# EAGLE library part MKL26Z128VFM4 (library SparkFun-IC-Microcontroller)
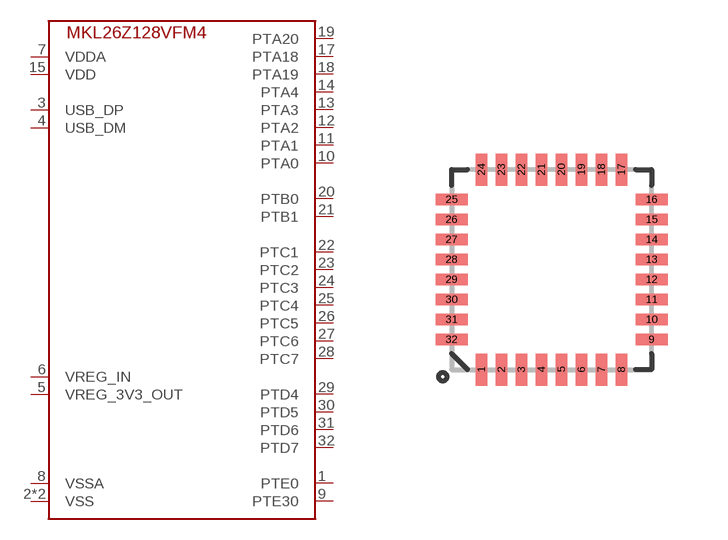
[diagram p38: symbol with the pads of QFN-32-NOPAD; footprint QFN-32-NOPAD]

Designator prefix -

## MKL26Z128VFM4 (PROD_ID: IC-15168)  [QFN-32-NOPAD]
1  PTE0
2  VSS
3  USB_DP
4  USB_DM
5  VREG_3V3_OUT
6  VREG_IN
7  VDDA
8  VSSA
9  PTE30
10  PTA0
11  PTA1
12  PTA2
13  PTA3
14  PTA4
15  VDD
16  VSS
17  PTA18
18  PTA19
19  PTA20
20  PTB0
21  PTB1
22  PTC1
23  PTC2
24  PTC3
25  PTC4
26  PTC5
27  PTC6
28  PTC7
29  PTD4
30  PTD5
31  PTD6
32  PTD7

## Footprint QFN-32-NOPAD (pad centres in mm)
QFN 32-Pin package w/ Thermal Pad ***Unproven*** Applicable Parts: TLC5940
smd 0.285 x 0.8: 1 -1.75,-2.5; 2 -1.25,-2.5; 3 -0.75,-2.5; 4 -0.25,-2.5; 5 0.25,-2.5; 6 0.75,-2.5; 7 1.25,-2.5; 8 1.75,-2.5; 17 1.75,2.5; 18 1.25,2.5; 19 0.75,2.5; 20 0.25,2.5; 21 -0.25,2.5; 22 -0.75,2.5; 23 -1.25,2.5; 24 -1.75,2.5
smd 0.8 x 0.285: 9 2.5,-1.75; 10 2.5,-1.25; 11 2.5,-0.75; 12 2.5,-0.25; 13 2.5,0.25; 14 2.5,0.75; 15 2.5,1.25; 16 2.5,1.75; 25 -2.5,1.75; 26 -2.5,1.25; 27 -2.5,0.75; 28 -2.5,0.25; 29 -2.5,-0.25; 30 -2.5,-0.75; 31 -2.5,-1.25; 32 -2.5,-1.75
